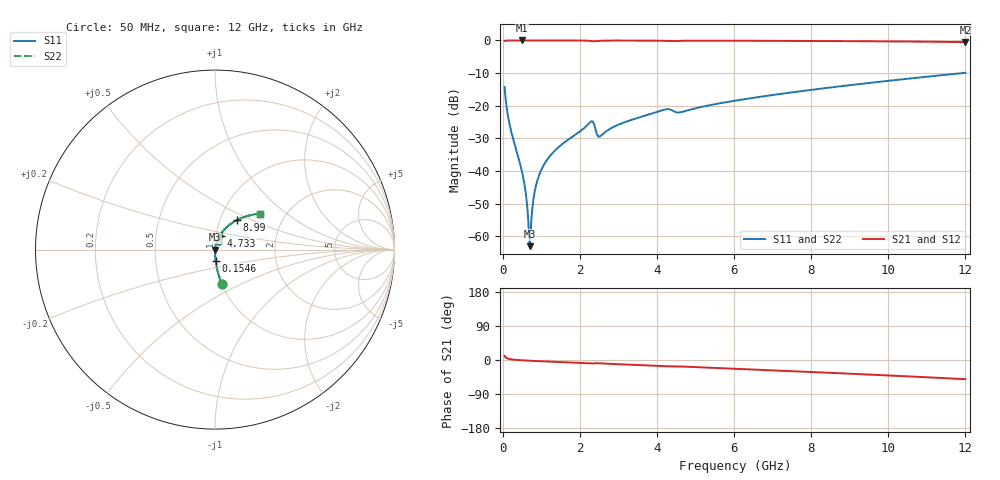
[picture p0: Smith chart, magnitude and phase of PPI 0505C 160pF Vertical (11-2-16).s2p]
# GHz S MA R 50
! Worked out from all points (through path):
!   1601 points, 50 MHz to 12 GHz, reference 50 ohm
!   highest |S21| = -0.01 dB at 505.6 MHz (marker M1); lowest = -0.5 dB at 12 GHz (marker M2)
!   group delay of S21, straight-line fit = 11.8 ps
!   lowest |S11| = -63.0 dB at 699.8 MHz (marker M3), VSWR 1.00, Z = 50.1 - j0.0122 ohm
!   |S11| at or under -10 dB: start of sweep to 11.92 GHz
!   |S22| runs from -63.0 to -9.9 dB; largest |S21 - S12| = 0
!   S11 on the Smith chart (normalised r, x): 50 MHz: 1.00, -0.40; 154.6 MHz: 1.00, -0.12; 4.733 GHz: 1.05, +0.16; 8.99 GHz: 1.20, +0.42; 12 GHz: 1.49, +0.66
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0.05  0.1939 -78.9  0.9808 11.0  0.9808 11.0  0.1939 -78.9
0.1545625  0.06104 -86.6  0.9977 3.1  0.9977 3.1  0.06104 -86.6
0.5055937  0.009511 -87.1  0.9993 -0.8  0.9993 -0.8  0.009511 -87.1
0.58775  0.005125 -84.0  0.9993 -1.3  0.9993 -1.3  0.005125 -84.0
0.6624375  0.001797 -69.2  0.9993 -1.7  0.9993 -1.7  0.001797 -69.2
0.6997813  0.0007101 -9.9  0.9993 -1.9  0.9993 -1.9  0.0007101 -9.9
0.737125  0.00156 60.4  0.9992 -2.1  0.9992 -2.1  0.00156 60.4
0.8043438  0.003961 76.7  0.9992 -2.4  0.9992 -2.4  0.003961 76.7
0.8640937  0.006026 79.9  0.9992 -2.7  0.9992 -2.7  0.006026 79.9
1.050812  0.01195 82.4  0.999 -3.6  0.999 -3.6  0.01195 82.4
1.394375  0.02175 82.3  0.9987 -5.1  0.9987 -5.1  0.02175 82.3
2.044156  0.0423 78.3  0.9962 -8.0  0.9962 -8.0  0.0423 78.3
2.305563  0.05786 60.4  0.9784 -9.4  0.9784 -9.4  0.05786 60.4
2.522156  0.03398 62.3  0.9883 -8.7  0.9883 -8.7  0.03398 62.3
3.015094  0.05173 75.9  0.9958 -11.2  0.9958 -11.2  0.05173 75.9
4.038312  0.08185 70.7  0.9912 -15.7  0.9912 -15.7  0.08185 70.7
4.732906  0.08302 67.4  0.989 -17.6  0.989 -17.6  0.08302 67.4
6.025  0.1196 65.5  0.9898 -23.2  0.9898 -23.2  0.1196 65.5
8.019156  0.1757 57.4  0.9812 -31.7  0.9812 -31.7  0.1757 57.4
8.990094  0.2063 53.2  0.9751 -36.1  0.9751 -36.1  0.2063 53.2
10.01331  0.2415 48.5  0.9667 -40.8  0.9667 -40.8  0.2415 48.5
12  0.3195 38.8  0.9432 -50.5  0.9432 -50.5  0.3195 38.8
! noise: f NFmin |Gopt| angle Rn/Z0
0.05  0.0003619  0.855  0.2761  0.0005329
1.372  0.00375  0.657  3.642  0.002084
2.701  0.01112  0.7586  7.281  0.009289
4.031  0.01442  0.7278  10.73  0.01045
5.36  0.01331  0.631  13.91  0.006677
6.682  0.01359  0.5686  16.77  0.005577
8.012  0.01528  0.5485  19.67  0.005873
9.341  0.01728  0.5401  22.53  0.006432
10.67  0.01949  0.5384  25.33  0.007153
12  0.02193  0.5418  28.09  0.008039
